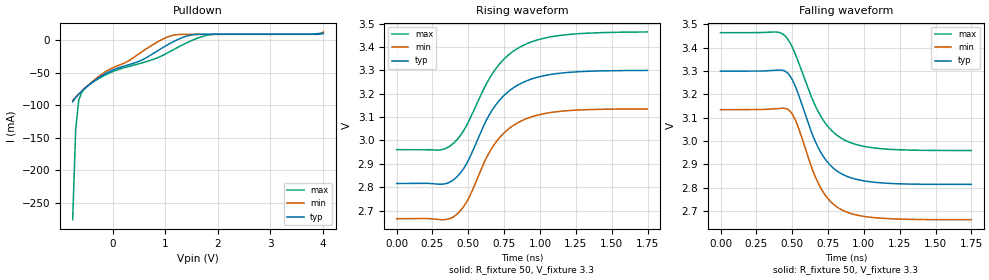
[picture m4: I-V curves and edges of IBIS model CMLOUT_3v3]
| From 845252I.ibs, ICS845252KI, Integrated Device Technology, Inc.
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[Model] CMLOUT_3v3
Model_type   Open_drain
Polarity   Non-Inverting
|   typ   min   max
C_comp   2pF   1.5pF   2.5pF
Vmeas = 3.095V
Rref = 50
Cref = 0
Vref = 3.3V
|   typ   min   max
[Voltage range]   3.3V   3.135V   3.465V
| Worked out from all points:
|   slope of the pulldown table from 0 to 0.495 V, typ, clamps not added: 37 ohm
|   rising waveform, R_fixture 50, V_fixture 3.3: 20-80 % time 269ps typ, 257ps min, 290ps max; typ from 2.82 V to 3.3 V
|   falling waveform, R_fixture 50, V_fixture 3.3: 20-80 % time 202ps typ, 190ps min, 224ps max; typ from 3.3 V to 2.81 V
[Pulldown]
|Voltage   I (typ)   I (min)   I (max)
|Note, modeling breaks down at 250mA and above.  This is well beyond the functional   |
|operating range of the device.  Should this scenario occur, catastrophic failure and   |
|possible damage to the device and/or board is of higher concern than the I-V curve   |
|behavior.  The IBIS checker will flag currents in excess of 10A with warnings.  Lines   |
|with currents in excess of 0.35 A have been commented out.  The points still remain|
|available to the user if the user desires to use them.   |
|-2.84000e+00   -7.27869e+00   -8.77380e+00   -5.95320e+00
|-2.38000e+00   -5.62014e+00   -6.67492e+00   -4.69424e+00
|-1.92000e+00   -3.95631e+00   -4.57058e+00   -3.43083e+00
|-1.46000e+00   -2.29232e+00   -2.47997e+00   -2.16371e+00
|-1.00000e+00   -6.61186e-01   -4.09748e-01   -9.13394e-01
|-9.90000e-01   -6.25854e-01   -3.64819e-01   -8.86724e-01
|-9.32644e-01   -4.23283e-01   -1.41941e-01   -7.33902e-01
|-8.75287e-01   -2.20871e-01   -1.06335e-01   -5.81264e-01
|-8.17931e-01   -1.11970e-01   -9.85647e-02   -4.28783e-01
-760.6mV  -94.66mA   -92.76mA   -276.5mA
-703.2mV  -87.98mA   -87.5mA    -136.9mA
-645.9mV  -82.77mA   -82.67mA   -92.27mA
-588.5mV  -78.11mA   -78.12mA   -80.15mA
-416.4mV  -66.29mA   -65.39mA   -66.61mA
-14.94mV  -46.18mA   -42.79mA   -48.61mA
558.6mV   -30.1mA    -17.38mA   -34.59mA
1.132V    -2.853mA   7.695mA    -15.28mA
1.476V    8.211mA    9.394mA    -1.114mA
1.878V    9.68mA     9.401mA    9.042mA
3.885V    9.756mA    9.437mA    10.45mA
4.01V     10.68mA    13.12mA    12.62mA
| 4.52800e+00   3.89204e+00   5.96316e+00   2.79665e+00
| 5.04600e+00   9.25980e+00   1.28193e+01   6.82274e+00
| 5.56400e+00   1.46320e+01   1.96797e+01   1.08529e+01
| 6.08200e+00   2.00061e+01   2.65419e+01   1.48853e+01
| 6.60000e+00   2.53813e+01   3.34046e+01   1.89193e+01
[Ramp]
|   typ   min   max
dV/dt_r   0.292/0.27n   0.284/0.257n   0.303/0.291n
dV/dt_f   0.294/0.203n   0.286/0.191n   0.304/0.224n
R_load =   50.0000
[Rising Waveform]
R_fixture = 50
V_fixture = 3.3
V_fixture_min = 3.135
V_fixture_max = 3.465
C_fixture = 0.0p
| Time   typ   min   max
0s        2.816V     2.665V     2.96V
306.6ps   2.813V     2.661V     2.959V
409.9ps   2.838V     2.679V     2.996V
495.7ps   2.909V     2.745V     3.073V
618.4ps   3.077V     2.916V     3.233V
686.7ps   3.148V     2.988V     3.303V
777.8ps   3.208V     3.048V     3.365V
889.9ps   3.251V     3.089V     3.409V
1.179ns   3.29V      3.127V     3.452V
1.748ns   3.3V       3.135V     3.464V
[Falling Waveform]
R_fixture = 50
V_fixture = 3.3
V_fixture_min = 3.135
V_fixture_max = 3.465
C_fixture = 0.0p
| Time   typ   min   max
0s        3.3V       3.135V     3.465V
395.9ps   3.305V     3.14V      3.467V
476.5ps   3.286V     3.133V     3.43V
530.8ps   3.221V     3.078V     3.359V
634.1ps   3.039V     2.89V      3.189V
695.4ps   2.956V     2.803V     3.111V
776ps     2.89V      2.736V     3.044V
877.6ps   2.85V      2.696V     3.001V
1.14ns    2.82V      2.669V     2.967V
1.748ns   2.815V     2.664V     2.96V
